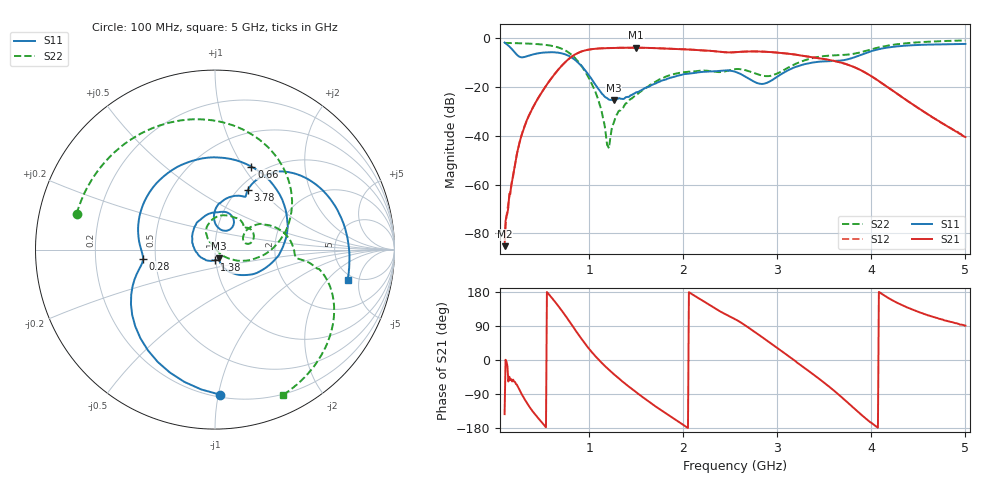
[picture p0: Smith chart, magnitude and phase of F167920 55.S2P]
!  2-Port S-parameters saved by WinCal
! VAR MeasName=S-Parameters (CALIBRATED_DATA) read from VNA (N5242A)
! VAR MeasDate=2016-11-22 9:58:13
! VAR NAME=F167920 55
! VAR FILENAME=F167920 55.S2P
! VAR DATE=2016-11-22 9:58:13
! VAR PHYS_PORTS=1,2
# Hz S DB R 50
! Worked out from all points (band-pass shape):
!   491 points, 100 MHz to 5 GHz, reference 50 ohm
!   highest |S21| = -3.93 dB at 1.5 GHz (marker M1); lowest = -85.3 dB at 100 MHz (marker M2)
!   |S21| within 3 dB of the highest: 840.6 MHz to 3.214 GHz (2.374 GHz wide, 117 % of centre)
!   lowest |S11| = -25.5 dB at 1.26 GHz (marker M3), VSWR 1.11, Z = 51.8 - j5.12 ohm
!   |S11| at or under -10 dB: 879.4 MHz to 3.378 GHz (2.499 GHz wide, 117 % of centre)
!   |S22| runs from -45.2 to -1.0 dB; largest |S21 - S12| = 0.00099
!   S11 on the Smith chart (normalised r, x): 100 MHz: 0.22, -1.01; 280 MHz: 0.43, -0.05; 660 MHz: 0.88, +1.09; 1.38 GHz: 0.99, -0.12; 3.78 GHz: 1.10, +0.86; 5 GHz: 4.36, -3.51
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1e8  -1.84 -88.0  -85.27 -142.9  -82.52 125.9  -1.98 165.5
1.7e8  -4.20 -136.1  -60.40 -50.6  -61.10 -56.2  -2.03 155.3
2.8e8  -7.88 -172.9  -39.86 -89.3  -39.93 -89.1  -2.14 138.6
4.5e8  -6.28 138.5  -25.07 -151.3  -25.05 -151.3  -2.47 110.2
5.6e8  -5.83 101.4  -18.47 176.5  -18.48 176.5  -2.91 88.6
6.6e8  -5.94 66.2  -13.41 146.0  -13.42 146.0  -3.72 65.4
7.8e8  -7.25 21.7  -8.64 105.1  -8.64 105.2  -5.89 32.2
9.2e8  -11.46 -29.1  -5.44 55.2  -5.43 55.2  -11.58 -7.7
1.09e9  -20.46 -66.3  -4.30 3.5  -4.29 3.5  -24.64 -37.5
1.2e9  -24.95 -67.8  -4.09 -23.7  -4.09 -23.8  -44.38 33.4
1.26e9  -25.46 -67.4  -4.05 -37.1  -4.04 -37.1  -34.74 111.7
1.38e9  -24.55 -91.3  -3.98 -62.0  -3.98 -62.0  -27.17 122.6
1.5e9  -22.20 -130.1  -3.93 -85.2  -3.92 -85.2  -23.28 122.0
1.74e9  -17.98 167.2  -4.18 -128.5  -4.18 -128.5  -17.08 107.4
2.08e9  -14.48 113.0  -4.73 175.8  -4.73 175.8  -13.70 63.8
2.55e9  -13.77 61.0  -5.78 108.1  -5.79 108.0  -12.73 27.4
2.82e9  -18.76 67.0  -5.51 63.6  -5.52 63.6  -15.17 11.5
3.01e9  -15.57 91.5  -5.98 29.9  -5.99 29.8  -14.32 29.8
3.37e9  -10.04 71.3  -7.80 -35.8  -7.80 -35.8  -8.22 15.2
3.78e9  -8.37 61.2  -11.31 -119.4  -11.32 -119.4  -6.63 -6.3
4.19e9  -3.78 37.7  -20.54 162.3  -20.58 162.4  -3.00 -21.9
5e9  -2.40 -13.0  -40.53 90.7  -40.66 90.9  -0.97 -64.9
